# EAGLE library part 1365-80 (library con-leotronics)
DUAL ROW STRAIGHT HEADER 1364 SERIES. 1.27mm x 1.27mm. Without Fixing Post. SMT Source: http://www.leotronics.co.uk/Conexcon/Data%20Sheets/sec.%20A/1364ing.pdf
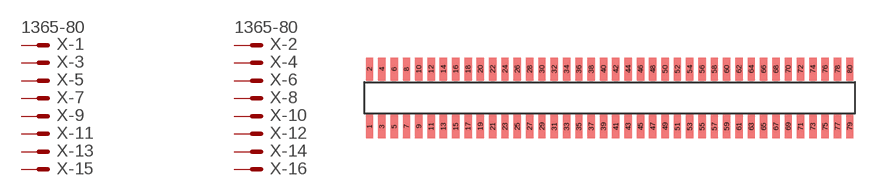
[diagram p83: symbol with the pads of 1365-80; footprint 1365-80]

Designator prefix X; gates -1=MVAL -2=MVAL -3=M -4=M -5=M -6=M -7=M -8=M -9=M -10=M -11=M -12=M -13=M -14=M -15=M -16=M -17=M -18=M -19=M -20=M -21=M -22=M -23=M -24=M -25=M -26=M -27=M -28=M -29=M -30=M -31=M -32=M -33=M -34=M -35=M -36=M -37=M -38=M -39=M -40=M -41=M -42=M -43=M -44=M -45=M -46=M -47=M -48=M -49=M -50=M -51=M -52=M -53=M -54=M -55=M -56=M -57=M -58=M -59=M -60=M -61=M -62=M -63=M -64=M -65=M -66=M -67=M -68=M -69=M -70=M -71=M -72=M -73=M -74=M -75=M -76=M -77=M -78=M -79=M -80=M

## 1365-80 (OC_FARNELL: unknown; OC_NEWARK: unknown)  [1365-80]
1  -1:S  pas
2  -2:S  pas
3  -3:S  pas
4  -4:S  pas
5  -5:S  pas
6  -6:S  pas
7  -7:S  pas
8  -8:S  pas
9  -9:S  pas
10  -10:S  pas
11  -11:S  pas
12  -12:S  pas
13  -13:S  pas
14  -14:S  pas
15  -15:S  pas
16  -16:S  pas
17  -17:S  pas
18  -18:S  pas
19  -19:S  pas
20  -20:S  pas
21  -21:S  pas
22  -22:S  pas
23  -23:S  pas
24  -24:S  pas
25  -25:S  pas
26  -26:S  pas
27  -27:S  pas
28  -28:S  pas
29  -29:S  pas
30  -30:S  pas
31  -31:S  pas
32  -32:S  pas
33  -33:S  pas
34  -34:S  pas
35  -35:S  pas
36  -36:S  pas
37  -37:S  pas
38  -38:S  pas
39  -39:S  pas
40  -40:S  pas
41  -41:S  pas
42  -42:S  pas
43  -43:S  pas
44  -44:S  pas
45  -45:S  pas
46  -46:S  pas
47  -47:S  pas
48  -48:S  pas
49  -49:S  pas
50  -50:S  pas
51  -51:S  pas
52  -52:S  pas
53  -53:S  pas
54  -54:S  pas
55  -55:S  pas
56  -56:S  pas
57  -57:S  pas
58  -58:S  pas
59  -59:S  pas
60  -60:S  pas
61  -61:S  pas
62  -62:S  pas
63  -63:S  pas
64  -64:S  pas
65  -65:S  pas
66  -66:S  pas
67  -67:S  pas
68  -68:S  pas
69  -69:S  pas
70  -70:S  pas
71  -71:S  pas
72  -72:S  pas
73  -73:S  pas
74  -74:S  pas
75  -75:S  pas
76  -76:S  pas
77  -77:S  pas
78  -78:S  pas
79  -79:S  pas
80  -80:S  pas

## Footprint 1365-80 (pad centres in mm)
DUAL ROW STRAIGHT HEADER 1364 SERIES. 1.27mm x 1.27mm. Without Fixing Post. SMT Source: http://www.leotronics.co.uk/Conexcon/Data%20Sheets/sec.%20A/1364ing.pdf
smd 0.76 x 2.4: 1 -24.765,-2.95; 2 -24.765,2.95; 3 -23.495,-2.95; 4 -23.495,2.95; 5 -22.225,-2.95; 6 -22.225,2.95; 7 -20.955,-2.95; 8 -20.955,2.95; 9 -19.685,-2.95; 10 -19.685,2.95; 11 -18.415,-2.95; 12 -18.415,2.95; 13 -17.145,-2.95; 14 -17.145,2.95; 15 -15.875,-2.95; 16 -15.875,2.95; 17 -14.605,-2.95; 18 -14.605,2.95; 19 -13.335,-2.95; 20 -13.335,2.95; 21 -12.065,-2.95; 22 -12.065,2.95; 23 -10.795,-2.95; 24 -10.795,2.95; 25 -9.525,-2.95; 26 -9.525,2.95; 27 -8.255,-2.95; 28 -8.255,2.95; 29 -6.985,-2.95; 30 -6.985,2.95; 31 -5.715,-2.95; 32 -5.715,2.95; 33 -4.445,-2.95; 34 -4.445,2.95; 35 -3.175,-2.95; 36 -3.175,2.95; 37 -1.905,-2.95; 38 -1.905,2.95; 39 -0.635,-2.95; 40 -0.635,2.95; 41 0.635,-2.95; 42 0.635,2.95; 43 1.905,-2.95; 44 1.905,2.95; 45 3.175,-2.95; 46 3.175,2.95; 47 4.445,-2.95; 48 4.445,2.95; 49 5.715,-2.95; 50 5.715,2.95; 51 6.985,-2.95; 52 6.985,2.95; 53 8.255,-2.95; 54 8.255,2.95; 55 9.525,-2.95; 56 9.525,2.95; 57 10.795,-2.95; 58 10.795,2.95; 59 12.065,-2.95; 60 12.065,2.95; 61 13.335,-2.95; 62 13.335,2.95; 63 14.605,-2.95; 64 14.605,2.95; 65 15.875,-2.95; 66 15.875,2.95; 67 17.145,-2.95; 68 17.145,2.95; 69 18.415,-2.95; 70 18.415,2.95; 71 19.685,-2.95; 72 19.685,2.95; 73 20.955,-2.95; 74 20.955,2.95; 75 22.225,-2.95; 76 22.225,2.95; 77 23.495,-2.95; 78 23.495,2.95; 79 24.765,-2.95; 80 24.765,2.95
